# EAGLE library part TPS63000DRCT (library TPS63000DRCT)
TPS63000DRCT Buck/Boost Converter, 1.2A, Adjustable, 1.2 5.5 V, 1500 kHz, 10-Pin SON EP Source: Datasheet
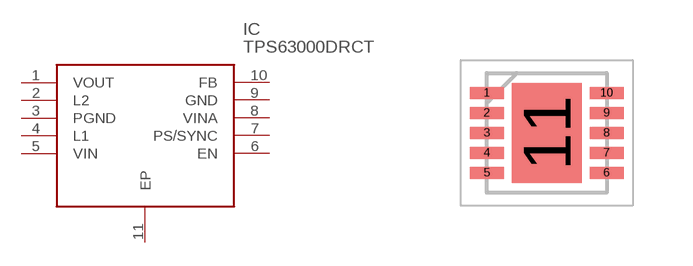
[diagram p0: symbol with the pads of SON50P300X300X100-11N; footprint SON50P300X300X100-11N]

Designator prefix IC

## TPS63000DRCT (Arrow_Part_Number: TPS63000DRCT; Arrow_Price/Stock: https://www.arrow.com/en/products/tps63000drct/texas-instruments; Description: TPS63000DRCT Buck/Boost Converter, 1.2A, Adjustable, 1.2 5.5 V, 1500 kHz, 10-Pin SON EP; Height: 1mm; Manufacturer_Name: Texas Instruments; Manufacturer_Part_Number: TPS63000DRCT; RS_Part_Number: 0389334P; RS_Price/Stock: http://uk.rs-online.com/web/p/products/0389334P)  [SON50P300X300X100-11N]
1  VOUT  out
2  L2
3  PGND  pwr
4  L1
5  VIN  in
6  EN
7  PS/SYNC
8  VINA  in
9  GND  pwr
10  FB
11  EP

## Footprint SON50P300X300X100-11N (pad centres in mm)
10-Pin QFN
smd 0.85 x 0.3: 1 -1.5,1; 2 -1.5,0.5; 3 -1.5,0; 4 -1.5,-0.5; 5 -1.5,-1; 6 1.5,-1; 7 1.5,-0.5; 8 1.5,0; 9 1.5,0.5; 10 1.5,1
smd 1.75 x 2.5: 11 0,0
